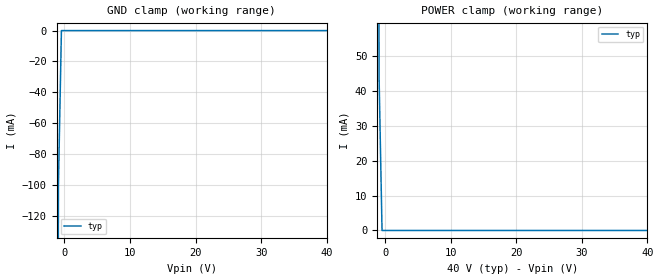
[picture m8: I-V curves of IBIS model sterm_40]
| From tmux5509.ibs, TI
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| sterm_40
[Model]   sterm_40
Model_type   Terminator
|   typ   min   max
C_comp   2.533030e-12   NA   NA
[Voltage Range]   40   NA   NA
[Temperature Range]   27   NA   NA
[Power Clamp Reference]   40   NA   NA
[GND Clamp Reference]   0   NA   NA
[GND Clamp]
|   Voltage   I(typ)   I(min)   I(max)
-5V       -13.02A    NA         NA
-1.364V   -1.178A    NA         NA
-909.1mV  -99.73mA   NA         NA
-454.5mV  -820.3nA   NA         NA
40V       660nA      NA         NA
[POWER Clamp]
|   Voltage   I(typ)   I(min)   I(max)
-5V       6.669A     NA         NA
-1.364V   578.8mA    NA         NA
-909.1mV  44.15mA    NA         NA
-454.5mV  512.2nA    NA         NA
40V       -3.008nA   NA         NA
